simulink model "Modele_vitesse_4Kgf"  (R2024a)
settings: Solver=VariableStepAuto  StartTime=0.0  StopTime=10  RelTol=1e-3
libraries: fl_lib x16, nesl_utility x7, simulink x1, ee_lib x1

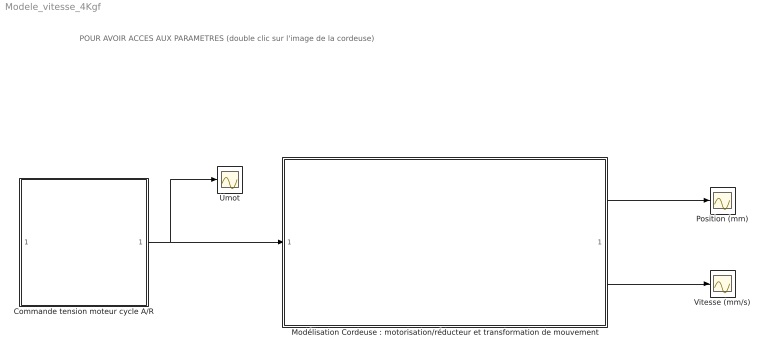
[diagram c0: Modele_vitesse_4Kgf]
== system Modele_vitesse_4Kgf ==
  note: POUR AVOIR ACCES AUX PARAMETRES (double clic sur l'image de la cordeuse)
  Commande tension moteur cycle A/R : Subsystem
  "Modélisation Cordeuse : motorisation/réducteur et transformation de mouvement" : Subsystem  mask{R=1.1, L=1, Ke=0.00262, Kred=50, Rp=8, f=0.00008, J=0.00012, Cr=0.0011}
      mask prompts: R "R en Ohms"; L "L en mH"; Ke "Ke en V/tr/min"; Kred "Rapport de réduction"; Rp "Rayon du pignon en mm"; f "Frottement visqueux N.m/(rad/s)"; J "Inertie équivalente kg.m²"; Cr "Couple frottement sec N.m"
  Position (mm) : Scope
  Umot : Scope
  Vitesse (mm/s) : Scope
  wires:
  "Modélisation Cordeuse : motorisation/réducteur et transformation de mouvement"/1(P) -> Position (mm)/1
  "Modélisation Cordeuse : motorisation/réducteur et transformation de mouvement"/2(V) -> Vitesse (mm/s)/1
  Commande tension moteur cycle A/R/1(Out1) -> Umot/1, "Modélisation Cordeuse : motorisation/réducteur et transformation de mouvement"/1(U)

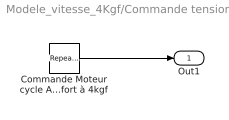
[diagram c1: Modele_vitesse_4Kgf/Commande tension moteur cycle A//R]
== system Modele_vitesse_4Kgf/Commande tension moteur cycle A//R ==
  Commande Moteur cycle A/R réglage effort à 4kgf : simulink/Sources/Repeating Sequence Interpolated  OutValues=[0 6.5 6.5 -13 -13 0 0].'  TimeValues=[0 0.01 3.5 3.51 5.25 5.26 100].'  LookUpMeth=Interpolation-Use End Values  tsamp=0.01  OutMin=[]  OutMax=[]  OutDataTypeStr=double  OutputDataTypeScalingMode=double  OutDataType=fixdt(0,8)  OutScaling=2^-10
  Out1 : Outport
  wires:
  Commande Moteur cycle A/R réglage effort à 4kgf/1 -> Out1/1

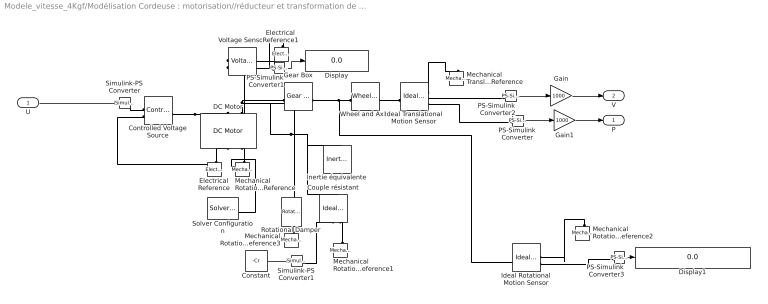
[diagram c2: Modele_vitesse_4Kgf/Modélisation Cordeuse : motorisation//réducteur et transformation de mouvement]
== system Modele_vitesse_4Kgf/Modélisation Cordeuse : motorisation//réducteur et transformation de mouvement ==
  U : Inport
  Constant : Constant  Value=-Cr
  Controlled Voltage Source : fl_lib/Electrical/Electrical Sources/Controlled Voltage Source
  Couple résistant : fl_lib/Mechanical/Mechanical Sources/Ideal Torque Source
  DC Motor : ee_lib/Electromechanical/Brushed Motors/DC Motor  field_option=ee.enum.field_option.pm  Rf=100 Ohm  Lf=1 H  Laf=0.15 H  If0=0 A  parameterization=ee.enum.dcparam_option.circuit_param  Ra=R Ohm  La=L mH  emf_or_torque=ee.enum.emf_or_torque.kv  Kv=Ke V/rpm  Ki=6.876e-4 N*m/A  T_stall=0.24e-3 N*m  w_max=19100 rpm  w_rated=15000 rpm  P_rated=0.08 W  V_rated=1.5 V  lam_param=ee.enum.lam_param.damping  i_noload=0 A  V_i_noload=1.5 V  J=0.01 cm^2*g  lam=0 N*m*s/rad  speed0=0 rpm  enable_fault_armature=simscape.enum.onoff.off  rev_faulted=1 / 3  G_faulted_armature=1e-5 S  fault_trigger_armature=ee.enum.faults.faultTrigger.temporal  t_fault_armature=1 s  max_permissible_current_armature=inf A  t_fail_on_current_armature=1 s  enable_fault_field=simscape.enum.onoff.off  G_faulted_field=1e-5 S  fault_trigger_field=ee.enum.faults.faultTrigger.temporal  t_fault_field=1 s  max_permissible_current_field=inf A  t_fail_on_current_field=1 s  fault_action=simscape.enum.assert.action.none  alpha=3.93e-3 1/K  Tmeas=25 degC  thermal_mass=100 J/K  initial_temperature=25 degC
  Display : Display
  Display1 : Display
  Electrical Reference : fl_lib/Electrical/Electrical Elements/Electrical Reference
  Electrical Reference1 : fl_lib/Electrical/Electrical Elements/Electrical Reference
  Gain : Gain  Gain=1000
  Gain1 : Gain  Gain=1000
  Gear Box : fl_lib/Mechanical/Mechanisms/Gear Box  ratio=Kred  t_in_specify=off  t_in_priority=None  t_in=0 N*m  t_in_nominal_specify=off  t_in_nominal_value=1  t_in_nominal_unit=N*m  t_out_specify=off  t_out_priority=None  t_out=0 N*m  t_out_nominal_specify=off  t_out_nominal_value=1  t_out_nominal_unit=N*m
  Ideal Rotational Motion Sensor : fl_lib/Mechanical/Mechanical Sensors/Ideal Rotational Motion Sensor  reference=foundation.enum.MeasurementReference.difference  acceleration_port=false  velocity_port=true  position_port=false  wrap_angle=false  offset=0 rad
  Ideal Translational Motion Sensor : fl_lib/Mechanical/Mechanical Sensors/Ideal Translational Motion Sensor  reference=foundation.enum.MeasurementReference.difference  acceleration_port=false  velocity_port=true  position_port=true  offset=0 mm
  Inertie équivalente : fl_lib/Mechanical/Rotational Elements/Inertia  inertia=J kg*m^2  num_ports=foundation.enum.numPorts2.one  w_specify=off  w_priority=High  w=0 rad/s  w_nominal_specify=off  w_nominal_value=1  w_nominal_unit=rad/s  t_specify=off  t_priority=None  t=0 N*m  t_nominal_specify=off  t_nominal_value=1  t_nominal_unit=N*m
  Mechanical Rotational Reference{,1..3} (4 alike) : fl_lib/Mechanical/Rotational Elements/Mechanical Rotational Reference
  Mechanical Translational Reference : fl_lib/Mechanical/Translational Elements/Mechanical Translational Reference
  PS-Simulink Converter{,1..3} (4 alike) : nesl_utility/PS-Simulink Converter  PhysicalDomain=network_engine_domain  SubClassName=ps_output  LeftPortType=input  RightPortType=output  PseudoPeriodic=off  Frequencies=[]  VectorFormat=inherit  Unit=inherit  AffineConversion=off
  Rotational Damper : fl_lib/Mechanical/Rotational Elements/Rotational Damper  D=f N*m*s/rad  w_specify=off  w_priority=None  w=0 rad/s  w_nominal_specify=off  w_nominal_value=1  w_nominal_unit=rad/s  t_specify=off  t_priority=None  t=0 N*m  t_nominal_specify=off  t_nominal_value=1  t_nominal_unit=N*m
  Simulink-PS Converter : nesl_utility/Simulink-PS Converter  PhysicalDomain=network_engine_domain  SubClassName=ps_input  LeftPortType=input  RightPortType=output  PseudoPeriodic=off  Frequencies=[]  NoiseDistribution=none  NoiseParameters=[]  Unit=1  AffineConversion=off  FilteringAndDerivatives=provide  SimscapeFilterOrder=1  InputFilterTimeConstant=0.001  UdotUserProvided=0
  Simulink-PS Converter1 : nesl_utility/Simulink-PS Converter  PhysicalDomain=network_engine_domain  SubClassName=ps_input  LeftPortType=input  RightPortType=output  PseudoPeriodic=off  Frequencies=[]  NoiseDistribution=none  NoiseParameters=[]  Unit=1  AffineConversion=off  FilteringAndDerivatives=provide  SimscapeFilterOrder=1  InputFilterTimeConstant=0.001  UdotUserProvided=0
  Solver Configuration : nesl_utility/Solver Configuration  PhysicalDomain=network_engine_domain  SubClassName=solver  LeftPortType=input  RightPortType=generic  Tones=[]  Harmonics=[]  SimulateNoise=off  Profile=off  UseLocalSampling=off  EnableSwitchedLinearOptims=on  FrequencyDomain=off  UseCCode=off  RelTol=0.001  AbsTol=0.001  MinStep=1e-09  ToWorkspace=off  RevertToSquareIcSolve=off  NumHomotopyIterations=100  PhasorMode=off  PhasorModeNumHarmonics=1  ConsistencySolver=NEWTON_XTOL_AFTER_FTOL  IndexReductionMethod=DerivativeReplacement  DoDC=off  ResidualTolerance=1e-09  ConsistencyTolSource=GLOBAL  ConsistencyAbsTol=0.001  ConsistencyRelTol=0.001  ConsistencyTolFactor=0.001  UseLocalSolver=off  LocalSolverChoice=NE_BACKWARD_EULER_ADVANCER  ResolveIndetEquations=on  FunctionEvalNumThread=1  LocalSolverSampleTime=0.001  DoFixedCost=off  MaxNonlinIter=3  MaxModeIter=2  ComputeImpulses=off  ImpulseIterations=2  LinearAlgebra=auto  LinearAlgebraNumThread=0  EquationFormulation=NE_TIME_EF  DelaysMemoryBudget=1024  AutomaticFiltering=on  FilteringTimeConstant=0.001  PartitionStorageMethod=AS_NEEDED  PartitionMemoryBudget=1024  PartitionMethod=ROBUST  MultibodyUseLocalSolver=off  MultibodyLocalSolverChoice=ODE1  MultibodyLocalSolverSampleTime=0.001
  Voltage Sensor : fl_lib/Electrical/Electrical Sensors/Voltage Sensor
  Wheel and Axle : fl_lib/Mechanical/Mechanisms/Wheel and Axle  R=Rp mm  or=1  t_specify=off  t_priority=None  t=0 N*m  t_nominal_specify=off  t_nominal_value=1  t_nominal_unit=N*m  f_specify=off  f_priority=None  f=0 N  f_nominal_specify=off  f_nominal_value=1  f_nominal_unit=N
  P : Outport
  V : Outport  Port=2
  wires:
  PS-Simulink Converter1/1 -> Display/1
  U/1 -> Simulink-PS Converter/1
  Constant/1 -> Simulink-PS Converter1/1
  PS-Simulink Converter3/1 -> Display1/1
  PS-Simulink Converter2/1 -> Gain/1
  Gain/1 -> V/1
  PS-Simulink Converter/1 -> Gain1/1
  Gain1/1 -> P/1
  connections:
  Simulink-PS Converter/RConn1 -- Controlled Voltage Source/RConn1
  Wheel and Axle/RConn1 -- Ideal Translational Motion Sensor/LConn1
  Wheel and Axle/LConn1 -- Ideal Rotational Motion Sensor/LConn1 -- Gear Box/RConn1
  DC Motor/LConn2 -- Rotational Damper/LConn1 -- Couple résistant/LConn1 -- Inertie équivalente/LConn1 -- Gear Box/LConn1
  Electrical Reference1/LConn1 -- Voltage Sensor/RConn2
  Mechanical Rotational Reference/LConn1 -- Solver Configuration/RConn1 -- DC Motor/RConn2
  Controlled Voltage Source/LConn1 -- DC Motor/LConn1 -- Voltage Sensor/LConn1
  Ideal Translational Motion Sensor/RConn1 -- Mechanical Translational Reference/LConn1
  Electrical Reference/LConn1 -- Controlled Voltage Source/RConn2 -- DC Motor/RConn1
  PS-Simulink Converter1/LConn1 -- Voltage Sensor/RConn1
  PS-Simulink Converter2/LConn1 -- Ideal Translational Motion Sensor/RConn2
  Mechanical Rotational Reference1/LConn1 -- Couple résistant/RConn2
  Simulink-PS Converter1/RConn1 -- Couple résistant/RConn1
  Mechanical Rotational Reference2/LConn1 -- Ideal Rotational Motion Sensor/RConn1
  PS-Simulink Converter3/LConn1 -- Ideal Rotational Motion Sensor/RConn2
  Ideal Translational Motion Sensor/RConn3 -- PS-Simulink Converter/LConn1
  Mechanical Rotational Reference3/LConn1 -- Rotational Damper/RConn1
